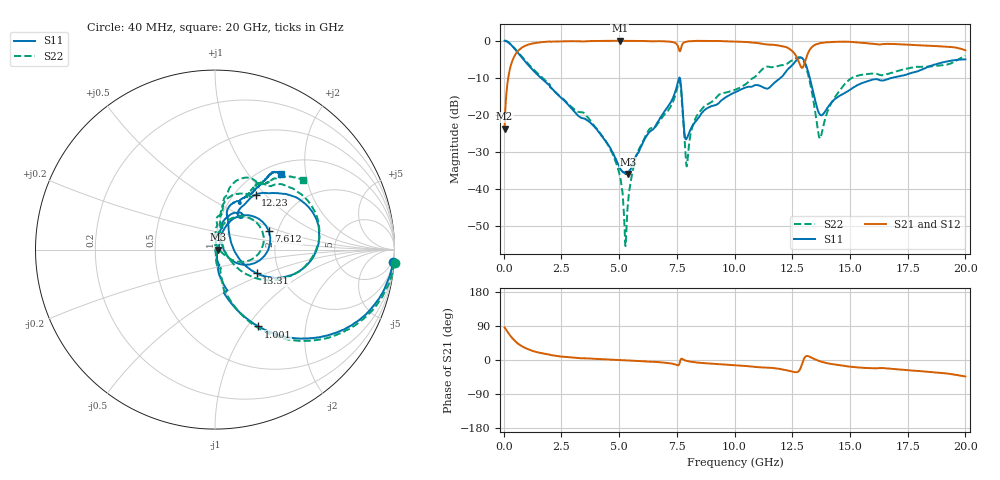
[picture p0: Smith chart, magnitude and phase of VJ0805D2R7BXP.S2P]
! VJ0805D2R7BXP
! DATE 10/29/2021  11:40
! CAPACITORS MOUNTED IN SERIES ON 25 MIL THICK MICROSTRIP SUBSTRATE
# GHz  S  MA  R  50.00
!  FREQ  S11M  S11A  S21M  S21A  S12M  S12A  S22M  S22A
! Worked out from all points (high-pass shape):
!   1601 points, 40 MHz to 20 GHz, reference 50 ohm
!   highest |S21| = -0.06 dB at 5.03 GHz (marker M1); lowest = -23.8 dB at 40 MHz (marker M2)
!   |S21| within 3 dB of the highest: 585 MHz to 12.54 GHz (11.95 GHz wide, 182 % of centre); 13.21 GHz to end of sweep
!   lowest |S11| = -36.1 dB at 5.379 GHz (marker M3), VSWR 1.03, Z = 51.6 + j0.00545 ohm
!   |S11| at or under -10 dB: 1.597 GHz to 7.61 GHz (6.013 GHz wide, 131 % of centre); 7.618 GHz to 12.01 GHz (4.391 GHz wide, 44.7 % of centre); 13.26 GHz to 16.86 GHz (3.601 GHz wide, 23.9 % of centre)
!   |S22| runs from -55.5 to 0.0 dB; largest |S21 - S12| = 0.0056
!   S11 on the Smith chart (normalised r, x): 40 MHz: 3, -29; 1.001 GHz: 1.00, -1.13; 7.612 GHz: 1.79, +0.41; 12.23 GHz: 1.24, +0.88; 13.31 GHz: 1.53, -0.43; 20 GHz: 1.19, +1.45
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0.04  0.9938 -4.0  0.06476 85.8  0.06797 84.7  1.004 -4.2
0.351875  0.8548 -30.6  0.5092 59.3  0.5091 59.3  0.8664 -30.9
1.000575  0.4913 -60.6  0.868 29.7  0.8671 29.7  0.5083 -60.5
3.370825  0.09004 -74.7  0.9737 4.6  0.9737 4.5  0.1077 -73.1
4.493575  0.04049 -73.3  0.9916 1.4  0.9912 1.4  0.03991 -84.1
5.03  0.01898 -48.4  0.9936 -0.2  0.9905 -0.2  0.01495 -75.4
5.25455  0.016 -19.2  0.9913 -0.9  0.9894 -1.0  0.002068 -41.7
5.3793  0.01575 0.2  0.9903 -1.3  0.9886 -1.3  0.006043 68.6
5.7785  0.02905 39.6  0.988 -2.5  0.9865 -2.6  0.03026 84.9
6.70165  0.08168 64.9  0.982 -5.6  0.9805 -5.6  0.0775 79.9
7.612325  0.3168 19.1  0.7324 -9.8  0.7314 -9.9  0.2827 21.5
7.94915  0.04916 34.6  0.9701 -2.7  0.9696 -2.8  0.02189 53.2
8.44815  0.09101 73.8  0.9915 -7.2  0.9897 -7.3  0.105 87.0
10.02  0.199 68.2  0.968 -13.6  0.9669 -13.7  0.2164 79.1
12.22808  0.3808 53.5  0.8181 -26.6  0.8166 -26.7  0.4764 48.3
12.90173  0.5864 8.1  0.4313 -14.9  0.431 -14.9  0.5827 5.4
13.3134  0.2672 -29.6  0.7924 7.0  0.7909 6.7  0.2312 -37.7
13.35083  0.24 -29.8  0.8163 5.8  0.815 5.5  0.2011 -38.8
13.7126  0.09967 10.7  0.9247 -3.7  0.9232 -3.8  0.04762 26.2
14.9102  0.2079 71.7  0.965 -16.9  0.9634 -17.1  0.2841 77.2
16.68165  0.3046 63.2  0.9012 -22.7  0.9009 -22.8  0.3569 59.2
20  0.5583 49.0  0.737 -43.5  0.7364 -43.7  0.6257 38.5
